[IBIS Ver]   3.2
[File Name]   sprm458.ibs
[File Rev]   1.0
[Date]   November 3, 2003
[Source]   File originated at Texas Instruments
[Copyright]   (c) 2003, Texas Instruments Inc.
[Component]   r2812zhh
[Manufacturer] Texas Instruments
[Package]
| Variable   Typ   Min   Max
R_pkg   0.08821   0.00445   0.1444
L_pkg   2.312e-09   3.373e-10   3.933e-09
C_pkg   2.855e-13   1.279e-13   4.259e-13
[Pin] signal_name   model_name   R_pin   L_pin   C_pin
B2   VDDAIO   NC   0.09209  2.36e-09   2.324e-13
C2   ADCINB0   NC   0.08702  2.145e-09  2.491e-13
C3   ADCINB1   NC   0.08455  2.129e-09  2.412e-13
B1   ADCINB2   NC   0.1237   3.291e-09  3.802e-13
C1   ADCINB3   NC   0.103   2.673e-09  3.339e-13
D3   ADCINB4   NC   0.07884  2.005e-09  2.389e-13
D2   ADCINB5   NC   0.07849  1.946e-09  2.548e-13
D1   ADCINB6   NC   0.09972  2.597e-09  2.918e-13
F5   ADCINB7   NC   0.1392   3.811e-09  4.225e-13
E4   ADCREFM   NC   0.1002   2.62e-09   3.512e-13
E2   ADCREFP   NC   0.07253  1.807e-09  2.304e-13
E3   AVSSREFBG   NC   0.07152  1.838e-09  2.399e-13
E1   AVDDREFBG   NC   0.09207  2.431e-09  2.756e-13
F4   VDDA1   NC   0.09478  2.501e-09  3.059e-13
F3   VSSA1   NC   0.06871  1.775e-09  2.4e-13
F2   ADCRESEXT   NC   0.06839  1.711e-09  2.218e-13
F1   XMPNMC   IDG09_PE100   0.09079  2.383e-09  2.69e-13
G5   XA(0)   OUI83   0.1124   3.004e-09  3.787e-13
G4   VSS   NC   0.09241  2.449e-09  3.276e-13
G2   MDRA   IDG09_OUO43_PS100  0.06703  1.677e-09  2.109e-13
G3   XD(0)   IDG09_OUI83_PS100  0.06663  1.72e-09   2.244e-13
G1   MDXA   IDG09_OUO43   0.08649  2.3e-09   3.064e-13
H1   VDD   NC   0.08687  2.308e-09  3.051e-13
H3   XD(1)   IDG09_OUI83_PS100  0.0675   1.739e-09  2.278e-13
H2   MCLKRA   IDG09_OUO43_PS100  0.06857  1.71e-09   2.172e-13
H4   MFSXA   IDG09_OUO43_PS100  0.0958   2.514e-09  3.319e-13
H5   XD(2)   IDG09_OUI83_PS100  0.1148   3.076e-09  3.819e-13
J1   MCLKXA   IDG09_OUO43_PS100  0.09444  2.462e-09  2.835e-13
J2   MFSRA   IDG09_OUO43_PS100  0.07272  1.804e-09  2.338e-13
J3   XD(3)   IDG09_OUI83_PS100  0.07371  1.889e-09  2.436e-13
J4   VDDIO   NC   0.09822  2.576e-09  3.054e-13
K1   VSS   NC   0.09654  2.518e-09  2.844e-13
K3   XD(4)   IDG09_OUI83_PS100  0.07688  1.955e-09  2.515e-13
K2   SPICLKA   IDG09_OUO43   0.07656  1.898e-09  2.333e-13
K4   SPISTEA   IDG09_OUO43   0.1045   2.711e-09  3.594e-13
J5   XD(5)   IDG09_OUI83_PS100  0.1444   3.933e-09  4.259e-13
L1   VDD   NC   0.1023   2.666e-09  2.93e-13
L2   VSS   NC   0.08196  2.025e-09  2.536e-13
L3   XD(6)   IDG09_OUI83_PS100  0.08003  2.035e-09  2.292e-13
M1   SPISIMOA   IDG09_OUO43   0.1022   2.66e-09   3.169e-13
N1   SPISOMIA   IDG09_OUO43   0.1206   3.247e-09  3.719e-13
M3   XRDn   OUI83   0.08199  2.072e-09  2.38e-13
M2   XA(1)   OUI83   0.08514  2.104e-09  2.563e-13
P1   XZCS0AND1n   OUI83   0.1272   3.432e-09  3.17e-13
N2   PWM7   IDG09_OUO43_PS100  0.09249  2.375e-09  2.344e-13
P2   PWM8   IDG09_OUO43_PS100  0.1091   2.835e-09  3.24e-13
N3   PWM9   IDG09_OUO43_PS100  0.0847   2.1e-09   2.977e-13
P3   PWM10   IDG09_OUO43_PS100  0.1058   2.786e-09  3.224e-13
L4   PWM11   IDG09_OUO43_PS100  0.1017   2.696e-09  3.056e-13
M4   PWM12   IDG09_OUO43_PS100  0.07819  1.991e-09  2.576e-13
N4   XRNW   OUI83   0.07522  1.886e-09  2.531e-13
P4   VSS   NC   0.09848  2.623e-09  3.028e-13
K5   T3PWM_T3CMP   IDG09_OUO43_PS100  0.1128   3.022e-09  3.435e-13
L5   XD(7)   IDG09_OUI83_PS100  0.09136  2.382e-09  3.006e-13
N5   T4PWM_T4CMP   IDG09_OUO43_PS100  0.06842  1.716e-09  2.385e-13
P5   VDD   NC   0.09175  2.499e-09  2.855e-13
M5   CAP4_QEP3   IDG09_OUO43_PS100  0.05893  1.5e-09   2.17e-13
K6   VSS   NC   0.1035   2.805e-09  3.409e-13
M6   CAP5_QEP4   IDG09_OUO43_PS100  0.06207  1.604e-09  2.311e-13
P6   CAP6_QEPI2   IDG09_OUO43_PS100  0.09133  2.468e-09  2.967e-13
N6   C4TRIPn   IDG09_OUO43_PS100  0.06341  1.612e-09  2.156e-13
L6   C5TRIPn   IDG09_OUO43_PS100  0.08399  2.26e-09   3.049e-13
K7   C6TRIPn   IDG09_OUO43_PS100  0.1038   2.828e-09  3.985e-13
L7   VDDIO   NC   0.08372  2.239e-09  3.16e-13
P7   XD(8)   IDG09_OUI83_PS100  0.0865   2.353e-09  2.75e-13
N7   TEST2   NC   0.06169  1.56e-09   2.049e-13
M7   TEST1   NC   0.06268  1.695e-09  2.38e-13
M8   XD(9)   IDG09_OUI83_PS100  0.06259  1.694e-09  2.398e-13
N8   VDDIO   NC   0.0611   1.546e-09  2.12e-13
P8   VSS   NC   0.08825  2.433e-09  2.701e-13
L8   TDIRB   IDG09_OUO43_PS100  0.08293  2.235e-09  3.129e-13
K8   TCLKINB   IDG09_OUO43_PS100  0.102   2.793e-09  3.815e-13
L9   XD(10)   IDG09_OUI83_PS100  0.0859   2.316e-09  3.071e-13
N9   XD(11)   IDG09_OUI83_PS100  0.06134  1.562e-09  2.256e-13
P9   VDD   NC   0.08678  2.402e-09  2.814e-13
M9   X2   NC   0.05751  1.488e-09  2.185e-13
K9   X1/XCLKIN   NC   0.1051   2.874e-09  3.416e-13
M10   VSS   NC   0.06466  1.77e-09   2.525e-13
P10   T3CTRIP_PDPINTBn IDG09_OUO43_PS100  0.09255  2.499e-09  2.906e-13
N10   XA(2)   OUI83   0.06746  1.702e-09  2.398e-13
L10   VDDIO   NC   0.09217  2.446e-09  3.236e-13
K10   XHOLDAn   OUI83   0.1143   3.12e-09   3.69e-13
P11   T4CTRIPn/EVBSOCn IDG09_OUO43_PS100  0.09684  2.574e-09  2.997e-13
N11   XWEn   OUI83   0.07403  1.857e-09  2.454e-13
M11   XA(3)   OUI83   0.07441  1.903e-09  2.389e-13
L11   VSS   NC   0.104   2.76e-09   3.07e-13
P12   VDD   NC   0.103   2.706e-09  3.157e-13
N12   CANTXA   IDG09_OUO43_PS100  0.08258  2.052e-09  2.669e-13
P13   XZCS2n   OUI83   0.1083   2.856e-09  2.829e-13
N13   CANRXA   IDG09_OUO43_PS100  0.09197  2.37e-09   2.499e-13
P14   SCITXDB   IDG09_OUO43   0.1255   3.388e-09  3.392e-13
M13   SCIRXDB   IDG09_OUO43   0.08237  2.039e-09  2.548e-13
M12   PWM1   IDG09_OUO43_PS100  0.08225  2.075e-09  2.456e-13
N14   VDDIO   NC   0.1201   3.231e-09  3.81e-13
M14   PWM2   IDG09_OUO43_PS100  0.09891  2.59e-09   3.294e-13
L12   PWM3   IDG09_OUO43_PS100  0.07898  2.006e-09  2.447e-13
L13   PWM4   IDG09_OUO43_PS100  0.07487  1.867e-09  2.444e-13
L14   XD(12)   IDG09_OUI83_PS100  0.09893  2.587e-09  2.886e-13
J10   XD(13)   IDG09_OUI83_PS100  0.1386   3.798e-09  4.176e-13
K11   PWM5   IDG09_OUO43_PS100  0.09954  2.607e-09  3.482e-13
K13   VSS   NC   0.0709   1.771e-09  2.325e-13
K12   VDD   NC   0.07034  1.811e-09  2.401e-13
K14   PWM6   IDG09_OUO43_PS100  0.09406  2.475e-09  2.775e-13
J11   T1PWM_T1CMP   IDG09_OUO43_PS100  0.09311  2.447e-09  3.027e-13
J12   XA(4)   OUI83   0.0707   1.815e-09  2.418e-13
J13   T2PWM_T2CMP   IDG09_OUO43_PS100  0.06707  1.681e-09  2.219e-13
J14   VSS   NC   0.09108  2.388e-09  2.791e-13
H10   CAP1_QEP1   IDG09_OUO43_PS100  0.1139   3.036e-09  3.844e-13
H11   CAP2_QEP2   IDG09_OUO43_PS100  0.09328  2.466e-09  3.308e-13
H13   XA(5)   OUI83   0.06503  1.629e-09  2.144e-13
H12   CAP3_QEPI1   IDG09_OUO43_PS100  0.06577  1.702e-09  2.25e-13
H14   T1CTRIP_PDPINTAn IDG09_OUO43_PS100  0.08639  2.297e-09  3.03e-13
G14   XA(6)   OUI83   0.0873   2.319e-09  3.041e-13
G12   VDD   NC   0.06918  1.777e-09  2.274e-13
G13   VSS   NC   0.06778  1.692e-09  2.146e-13
G11   VDDIO   NC   0.09314  2.459e-09  3.346e-13
G10   T2CTRIPn/EVASOCn IDG09_OUO43_PS100  0.1138   3.052e-09  3.802e-13
F14   TDIRA   IDG09_OUO43_PS100  0.09404  2.462e-09  2.798e-13
F13   TCLKINA   IDG09_OUO43_PS100  0.06786  1.696e-09  2.218e-13
F12   XA(7)   OUI83   0.07232  1.856e-09  2.474e-13
F11   XCLKOUT   OUI83   0.09426  2.507e-09  3.058e-13
E14   VSS   NC   0.09525  2.497e-09  2.91e-13
E12   XA(8)   OUI83   0.07626  1.938e-09  2.582e-13
E13   C1TRIPn   IDG09_OUO43_PS100  0.07579  1.878e-09  2.366e-13
E11   C2TRIPn   IDG09_OUO43_PS100  0.1028   2.672e-09  3.561e-13
F10   C3TRIPn   IDG09_OUO43_PS100  0.1414   3.864e-09  4.252e-13
D14   XA(9)   OUI83   0.1035   2.69e-09   2.981e-13
D13   TMS   IDG09_PS100   0.07795  1.936e-09  2.479e-13
D12   TDO   OUI83   0.08151  2.062e-09  2.503e-13
C14   VDD   NC   0.1046   2.725e-09  3.442e-13
B14   VSS   NC   0.1242   3.313e-09  3.855e-13
C12   XA(10)   OUI83   0.08905  2.226e-09  2.563e-13
C13   TDI   IDG09_PS100   0.0903   2.216e-09  2.631e-13
A14   XA(11)   OUI83   0.1281   3.455e-09  3.132e-13
B13   XZCS6AND7n   OUI83   0.09387  2.397e-09  2.377e-13
A13   TESTSEL   IDG09_PE100   0.1042   2.726e-09  3.249e-13
B12   TRSTn   IDG09_PE100   0.00445  3.373e-10  1.279e-13
A12   TCK   IDG09_PS100   0.1012   2.679e-09  3.184e-13
D11   EMU0   IDG09_OUI83_PS100  0.09979  2.649e-09  3.147e-13
C11   XA(12)   OUI83   0.07303  1.881e-09  2.526e-13
B11   XD(14)   IDG09_OUI83_PS100  0.07161  1.807e-09  2.388e-13
A11   XF_XPLLDIS   IDG09_OUI83_PS100  0.09603  2.567e-09  2.922e-13
E10   XA(13)   OUI83   0.1156   3.087e-09  3.455e-13
D10   VSS   NC   0.09186  2.405e-09  2.985e-13
B10   VDD   NC   0.06885  1.731e-09  2.29e-13
A10   XA(14)   OUI83   0.09485  2.561e-09  2.856e-13
C10   VSS   NC   0.063988 1.613e-09  2.243e-13
E9   VDDIO   NC   0.1082   2.906e-09  3.452e-13
C9   EMU1   IDG09_OUI83_PS100  0.06274  1.614e-09  2.346e-13
A9   XD(15)   IDG09_OUI83_PS100  0.09338  2.506e-09  3.182e-13
B9   XA(15)   OUI83   0.06408  1.62e-09   2.367e-13
D9   XINT1_XBIOn   IDG09_OUO43   0.08668  2.311e-09  3.397e-13
E8   XNMI_XINT13   IDG09_OUO43_PS100  0.1043   2.833e-09  3.974e-13
D8   XINT2_ADCSOC   IDG09_OUO43   0.08381  2.248e-09  3.111e-13
A8   XA(16)   OUI83   0.08698  2.367e-09  2.747e-13
B8   VSS   NC   0.06146  1.548e-09  2.203e-13
C8   VDD   NC   0.0627   1.691e-09  2.545e-13
C7   SCITXDA   IDG09_OUO43_PS100  0.06257  1.689e-09  2.491e-13
B7   XA(17)   OUI83   0.06157  1.552e-09  2.151e-13
A7   SCIRXDA   IDG09_OUO43_PS100  0.08827  2.43e-09   2.835e-13
D7   XA(18)   OUI83   0.08506  2.269e-09  3.34e-13
E7   XHOLDn   IDG09_PS100   0.1043   2.826e-09  3.994e-13
D6   XRSn   IDG09_OUM42_PS100  0.08576  2.305e-09  3.177e-13
B6   XREADY   IDG09_PS100   0.0641   1.621e-09  2.324e-13
A6   VDD1   NC   0.09005  2.472e-09  2.845e-13
C6   VSS1   NC   0.06117  1.569e-09  2.29e-13
E6   ADCBGREFIN   NC   0.1067   2.898e-09  3.505e-13
C5   VSSA2   NC   0.06463  1.768e-09  2.521e-13
A5   VDDA2   NC   0.09355  2.521e-09  2.935e-13
B5   ADCINA7   NC   0.06979  1.749e-09  2.589e-13
D5   ADCINA6   NC   0.09531  2.493e-09  3.268e-13
E5   ADCINA5   NC   0.115   3.131e-09  3.515e-13
A4   ADCINA4   NC   0.101   2.662e-09  3.031e-13
B4   ADCINA3   NC   0.07696  1.923e-09  2.515e-13
C4   ADCINA2   NC   0.0785   1.993e-09  2.483e-13
D4   ADCINA1   NC   0.1037   2.755e-09  3.086e-13
A3   ADCINA0   NC   0.1053   2.763e-09  3.109e-13
B3   ADCLO   NC   0.08665  2.149e-09  2.561e-13
A2   VSSAIO   NC   0.1087   2.841e-09  2.701e-13
| End of package information
|   GS30 Cell IDG09_PE100
|   Component IDG09_PE100
[Component]   IDG09_PE100
[Manufacturer]   Texas Instruments
[Package]
|  variable   typ   min   max
R_pkg   0   0   0
L_pkg   0   0   0
C_pkg   0   0   0
[Pin]   signal_name   model_name   R_pin   L_pin   C_pin
VDDS   VDDS   POWER
VSS   VSS   GND
PAD   PAD   IDG09_PE100
[Model Selector] IDG09_PE100
9_PE100_PULLDOWN_2P5  Cell operated at 2.5(nom)
|IDG09_PE100_PULLDOWN_2P5; BUFFER WITH WEAK_PULLDOWN_ON
PE100_NOPULLDOWN_2P5  Cell operated at 2.5(nom)
|IDG09_PE100_NOPULLDOWN_2P5; BUFFER OPERATING IN NORMMAL MODE WITHOUT PULLD
|OWN
9_PE100_PULLDOWN_3P3  Cell operated at 3.3(nom)
|IDG09_PE100_PULLDOWN_3P3; BUFFER WITH WEAK_PULLDOWN_ON
PE100_NOPULLDOWN_3P3  Cell operated at 3.3(nom)
|IDG09_PE100_NOPULLDOWN_3P3; BUFFER OPERATING IN NORMMAL MODE WITHOUT PULLD
|OWN
_PE100_PULLDOWN_2P75  Cell operated at 2.75(nom)
|IDG09_PE100_PULLDOWN_2P75; BUFFER WITH WEAK_PULLDOWN_ON
E100_NOPULLDOWN_2P75  Cell operated at 2.75(nom)
[Component]   IDG09_OUO43
[Manufacturer]   Texas Instruments
[Package]
|  variable   typ   min   max
R_pkg   0   0   0
L_pkg   0   0   0
C_pkg   0   0   0
[Pin]   signal_name   model_name   R_pin   L_pin   C_pin
VSS   VSS   GND
VDDS   VDDS   POWER
PAD   PAD   IDG09_OUO43
[Model Selector] IDG09_OUO43
IDG09_OUO43_2P5  Cell operated at 2.5(nom)
|IDG09_OUO43_2P5; DEFAULT
IDG09_OUO43_3P3  Cell operated at 3.3(nom)
|IDG09_OUO43_3P3; DEFAULT
IDG09_OUO43_2P75  Cell operated at 2.75(nom)
|   Component IDG09_PS100
[Component]   IDG09_PS100
[Manufacturer]   Texas Instruments
[Package]
|  variable   typ   min   max
R_pkg   0   0   0
L_pkg   0   0   0
C_pkg   0   0   0
[Pin]   signal_name   model_name   R_pin   L_pin   C_pin
VDDS   VDDS   POWER
VSS   VSS   GND
PAD   PAD   IDG09_PS100
[Model Selector] IDG09_PS100
G09_PS100_PULLUP_2P5  Cell operated at 2.5(nom)
|IDG09_PS100_PULLUP_2P5; BUFFER WITH WEAK_PULLUP_ON
9_PS100_NOPULLUP_2P5  Cell operated at 2.5(nom)
|IDG09_PS100_NOPULLUP_2P5; BUFFER OPERATING IN NORMMAL MODE WITHOUT PULLUP
G09_PS100_PULLUP_3P3  Cell operated at 3.3(nom)
|IDG09_PS100_PULLUP_3P3; BUFFER WITH WEAK_PULLUP_ON
9_PS100_NOPULLUP_3P3  Cell operated at 3.3(nom)
|IDG09_PS100_NOPULLUP_3P3; BUFFER OPERATING IN NORMMAL MODE WITHOUT PULLUP
09_PS100_PULLUP_2P75  Cell operated at 2.75(nom)
|IDG09_PS100_PULLUP_2P75; BUFFER WITH WEAK_PULLUP_ON
_PS100_NOPULLUP_2P75  Cell operated at 2.75(nom)
|   Component OUI83
[Component]   OUI83
[Manufacturer]   Texas Instruments
[Package]
|  variable   typ   min   max
R_pkg   0   0   0
L_pkg   0   0   0
C_pkg   0   0   0
[Pin]   signal_name   model_name   R_pin   L_pin   C_pin
VSS   VSS   GND
VDDS   VDDS   POWER
Y   Y   OUI83
[Model Selector] OUI83
OUI83_2P5  Cell operated at 2.5(nom)
|OUI83_2P5; DEFAULT
OUI83_3P3  Cell operated at 3.3(nom)
|OUI83_3P3; DEFAULT
OUI83_2P75  Cell operated at 2.75(nom)
|   Component IDG09_OUI83_PS100
[Component]   IDG09_OUI83_PS100
[Manufacturer]   Texas Instruments
[Package]
|  variable   typ   min   max
R_pkg   0   0   0
L_pkg   0   0   0
C_pkg   0   0   0
[Pin]   signal_name   model_name   R_pin   L_pin   C_pin
VSS   VSS   GND
VDDS   VDDS   POWER
PAD   PAD   IDG09_OUI83_PS100
[Model Selector] IDG09_OUI83_PS100
UI83_PS100_PU_ON_2P5  Cell operated at 2.5(nom)
|IDG09_OUI83_PS100_PU_ON_2P5; BUFFER WITH WEAK_PULLUP_ON
I83_PS100_PU_OFF_2P5  Cell operated at 2.5(nom)
|IDG09_OUI83_PS100_PU_OFF_2P5; BUFFER IN NORMAL MODE WITH PULLUP AND PUL
|LDOWN OFF
UI83_PS100_PU_ON_3P3  Cell operated at 3.3(nom)
|IDG09_OUI83_PS100_PU_ON_3P3; BUFFER WITH WEAK_PULLUP_ON
I83_PS100_PU_OFF_3P3  Cell operated at 3.3(nom)
|IDG09_OUI83_PS100_PU_OFF_3P3; BUFFER IN NORMAL MODE WITH PULLUP AND PUL
|LDOWN OFF
I83_PS100_PU_ON_2P75  Cell operated at 2.75(nom)
|IDG09_OUI83_PS100_PU_ON_2P75; BUFFER WITH WEAK_PULLUP_ON
83_PS100_PU_OFF_2P75  Cell operated at 2.75(nom)
|   Component IDG09_OUO43_PS100
[Component]   IDG09_OUO43_PS100
[Manufacturer]   Texas Instruments
[Package]
|  variable   typ   min   max
R_pkg   0   0   0
L_pkg   0   0   0
C_pkg   0   0   0
[Pin]   signal_name   model_name   R_pin   L_pin   C_pin
VSS   VSS   GND
VDDS   VDDS   POWER
PAD   PAD   IDG09_OUO43_PS100
[Model Selector] IDG09_OUO43_PS100
UO43_PS100_PU_ON_2P5  Cell operated at 2.5(nom)
|IDG09_OUO43_PS100_PU_ON_2P5; BUFFER WITH WEAK_PULLUP_ON
O43_PS100_PU_OFF_2P5  Cell operated at 2.5(nom)
|IDG09_OUO43O43_PS100_PU_OFF_2P5; BUFFER IN NORMAL MODE WITH PULLUP
| OFF
UO43_PS100_PU_ON_3P3  Cell operated at 3.3(nom)
|IDG09_OUO43_PS100_PU_ON_3P3; BUFFER WITH WEAK_PULLUP_ON
O43_PS100_PU_OFF_3P3  Cell operated at 3.3(nom)
|IDG09_OUO43_PS100_PU_OFF_3P3; BUFFER IN NORMAL MODE WITH PULLUP
| OFF
O43_PS100_PU_ON_2P75  Cell operated at 2.75(nom)
|IDG09_OUO43_PS100_PU_ON_2P75; BUFFER WITH WEAK_PULLUP_ON
43_PS100_PU_OFF_2P75  Cell operated at 2.75(nom)
|   Component IDG09_OUM42_PS100
[Component]   IDG09_OUM42_PS100
[Manufacturer]   Texas Instruments
[Package]
|  variable   typ   min   max
R_pkg   0   0   0
L_pkg   0   0   0
C_pkg   0   0   0
[Pin]   signal_name   model_name   R_pin   L_pin   C_pin
VSS   VSS   GND
VDDS   VDDS   POWER
PAD   PAD   IDG09_OUM42_PS100
[Model Selector] IDG09_OUM42_PS100
UM42_PS100_PU_ON_2P5  Cell operated at 2.5(nom)
|IDG09_OUM42_PS100_PU_ON_2P5; BUFFER WITH WEAK_PULLUP_ON
M42_PS100_PU_OFF_2P5  Cell operated at 2.5(nom)
|IDG09_OUM42_PS100_PU_OFF_2P5; BUFFER IN NORMAL MODE WITH PULLUP OFF
UM42_PS100_PU_ON_3P3  Cell operated at 3.3(nom)
|IDG09_OUM42_PS100_PU_ON_3P3; BUFFER WITH WEAK_PULLUP_ON
M42_PS100_PU_OFF_3P3  Cell operated at 3.3(nom)
|IDG09_OUM42_PS100_PU_OFF_3P3; BUFFER IN NORMAL MODE WITH PULLUP OFF
M42_PS100_PU_ON_2P75  Cell operated at 2.75(nom)
|IDG09_OUM42_PS100_PU_ON_2P75; BUFFER WITH WEAK_PULLUP_ON
42_PS100_PU_OFF_2P75  Cell operated at 2.75(nom)
| Models and submodels in the file (36): 9_PE100_PULLDOWN_2P5 (Input), PE100_NOPULLDOWN_2P5 (Input), 9_PE100_PULLDOWN_3P3 (Input), PE100_NOPULLDOWN_3P3 (Input), _PE100_PULLDOWN_2P75 (Input), E100_NOPULLDOWN_2P75 (Input), IDG09_OUO43_2P5 (I/O), IDG09_OUO43_3P3 (I/O), IDG09_OUO43_2P75 (I/O), G09_PS100_PULLUP_2P5 (Input), 9_PS100_NOPULLUP_2P5 (Input), G09_PS100_PULLUP_3P3 (Input), 9_PS100_NOPULLUP_3P3 (Input), 09_PS100_PULLUP_2P75 (Input), _PS100_NOPULLUP_2P75 (Input), OUI83_2P5 (3-state), OUI83_3P3 (3-state), OUI83_2P75 (3-state), UI83_PS100_PU_ON_2P5 (I/O), I83_PS100_PU_OFF_2P5 (I/O), UI83_PS100_PU_ON_3P3 (I/O), I83_PS100_PU_OFF_3P3 (I/O), I83_PS100_PU_ON_2P75 (I/O), 83_PS100_PU_OFF_2P75 (I/O), UO43_PS100_PU_ON_2P5 (I/O), O43_PS100_PU_OFF_2P5 (I/O), UO43_PS100_PU_ON_3P3 (I/O), O43_PS100_PU_OFF_3P3 (I/O), O43_PS100_PU_ON_2P75 (I/O), 43_PS100_PU_OFF_2P75 (I/O), UM42_PS100_PU_ON_2P5 (I/O_open_drain), M42_PS100_PU_OFF_2P5 (I/O_open_drain), UM42_PS100_PU_ON_3P3 (I/O_open_drain), M42_PS100_PU_OFF_3P3 (I/O_open_drain), M42_PS100_PU_ON_2P75 (I/O_open_drain), 42_PS100_PU_OFF_2P75 (I/O_open_drain)
